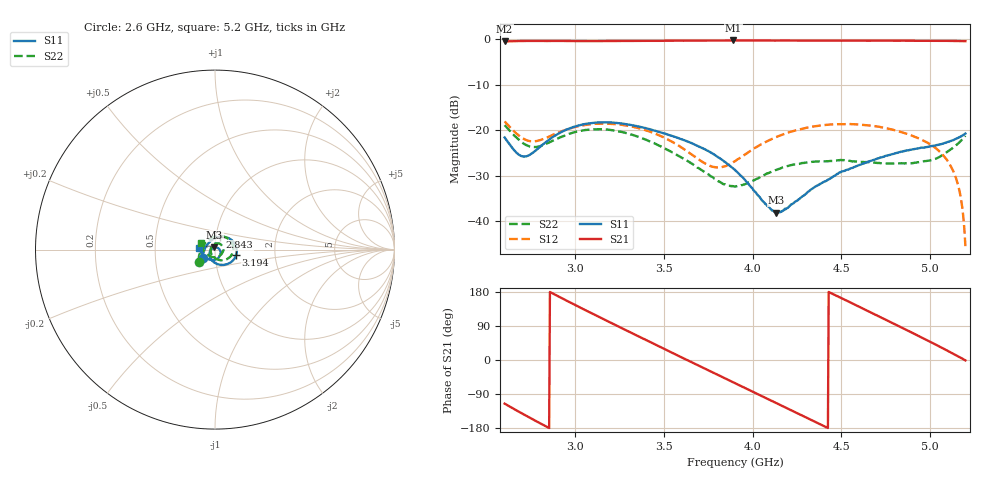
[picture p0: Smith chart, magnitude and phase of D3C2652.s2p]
! 11/4/2020 11:02:23 AM
! C:\USERS\DITOM\DESKTOP\SINGLE JUNCTION ISOLATOR DATA\2.6-5.2 GHZ (D3I2652).S2P
! CHANNEL.1
! TR.MEASUREMENT
! CORRECTED.DATA
# GHZ S RI R 50.0
! FREQ.GHZ  S11RE  S11IM  S21RE  S21IM  S12RE  S12IM  S22RE  S22IM
!; PortSelection: Port_12
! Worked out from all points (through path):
!   601 points, 2.6 GHz to 5.2 GHz, reference 50 ohm
!   highest |S21| = -0.24 dB at 3.891 GHz (marker M1); lowest = -0.5 dB at 2.6 GHz (marker M2)
!   lowest |S11| = -38.2 dB at 4.134 GHz (marker M3), VSWR 1.02, Z = 49.7 + j1.19 ohm
!   |S11| at or under -10 dB: start of sweep to end of sweep
!   |S22| runs from -32.4 to -18.9 dB; largest |S21 - S12| = 1
!   S11 on the Smith chart (normalised r, x): 2.6 GHz: 0.87, -0.08; 2.843 GHz: 1.05, +0.15; 3.194 GHz: 1.26, -0.08; 5.2 GHz: 0.83, +0.02
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2.6  -0.0695 -0.0455  -0.4025 -0.8588  -0.0272 0.1217  -0.0914 -0.0675
2.708333  -0.04 0.032  -0.7732 -0.5674  -0.00793 0.0796  -0.0681 0.0197
2.842667  0.0287 0.0705  -0.9586 -0.0437  -0.00673 0.0832  -0.00158 0.0718
3.037667  0.1104 0.0328  -0.688 0.6678  0.0677 0.0899  0.0871 0.0471
3.193667  0.1172 -0.0319  -0.1585 0.9447  0.1168 0.0137  0.0997 -0.0132
3.323667  0.0882 -0.0706  0.3336 0.8998  0.089 -0.0628  0.0733 -0.0493
3.466667  0.045 -0.0852  0.7683 0.5802  0.00725 -0.0882  0.0336 -0.0595
3.570667  0.0156 -0.0816  0.9416 0.2219  -0.0414 -0.0561  0.00902 -0.0527
3.679  -0.00977 -0.0678  0.9507 -0.1909  -0.0501 -0.00196  -0.0102 -0.0387
3.787333  -0.0264 -0.0461  0.7851 -0.5681  -0.016 0.0356  -0.0224 -0.0183
3.891333  -0.0309 -0.0216  0.4952 -0.8368  0.0317 0.0314  -0.0239 0.00368
3.9  -0.0306 -0.0199  0.4663 -0.853  0.0352 0.0289  -0.0233 0.00525
4.017  -0.0205 0.00226  0.0389 -0.971  0.0607 -0.0216  -0.0118 0.0262
4.134  -0.00292 0.0119  -0.3962 -0.8848  0.0322 -0.0777  0.00835 0.0356
4.337667  0.0223 0.00431  -0.912 -0.332  -0.0864 -0.0669  0.0388 0.0225
4.437333  0.0289 -0.00565  -0.9691 0.0418  -0.1153 -0.00512  0.0449 0.00904
4.545667  0.0314 -0.0204  -0.8641 0.4377  -0.0948 0.068  0.0452 -0.00846
4.766667  0.0115 -0.0518  -0.212 0.9419  0.0445 0.0936  0.0219 -0.037
4.927  -0.0244 -0.0577  0.3983 0.8783  0.0825 0.00498  -0.0135 -0.042
5.096  -0.0657 -0.0333  0.8711 0.4102  0.0173 -0.0437  -0.0559 -0.0135
5.161  -0.082 -0.0106  0.9462 0.1522  -0.00447 -0.0235  -0.0708 0.012
5.2  -0.0911 0.0103  0.9553 -0.0169  -0.00439 -0.00293  -0.0789 0.0355
